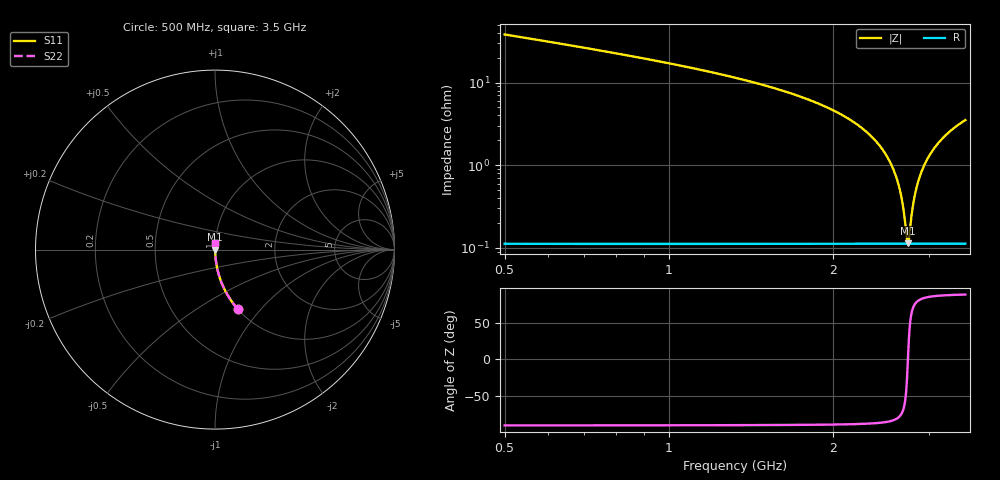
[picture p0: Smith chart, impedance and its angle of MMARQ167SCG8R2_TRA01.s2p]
! MMARQ167SCG8R2_TRA01  S-PARAMETER MODEL  ( General Type )
! Model Generated by TAIYO YUDEN Corporation (http://www.ty-top.com)
! Version 1.0
! TAIYO YUDEN Control No. 150305
! Copyright(c) 2015 TAIYO YUDEN CO.,LTD. All Rights Reserved.
! Product Description (link to TY-COMPAS)
! https://ds.yuden.co.jp/TYCOMPAS/or/detail?pn=MMARQ167SCG8R2CTRA01&u=M
! Products Name : Multilayer Ceramic Capacitors
! Characteristics :
!  Capacitance : 8.2 pF , Rated Voltage : 250V , TCC : CG / C0G
!  Case Size : 1.6 x 0.8 / 0.063 x 0.031 [mm/inch] , Thickness : 0.7 / 0.028 [mm/inch]
!  (Conditions: Temperature = 25 degC , DC Bias Current/Voltage = 0A / 0V)
! External Node Assignments :
!  1  o---| |---o  2
! GND o---------o GND
! Frequency Range : 500MHz  -  3.5GHz  [ 401 STEP ]
# MHz S RI R 50
! Freq[MHz].  S11 Real  S11 Imag  S21 Real  S21 Imag  S12 Real  S12 Imag  S22 Real  S22 Imag
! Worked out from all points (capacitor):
!   401 points, 500 MHz to 3.5 GHz, reference 50 ohm
!   read as one part in series: C = 8.06 pF near 515 MHz
!   lowest |Z| = 114 mohm at 2.743 GHz (marker M1)
!   series resonance near 2.746 GHz, so ESL is about 420 pH
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500  0.1281 -0.3327  0.8719 0.3327  0.8719 0.3327  0.1281 -0.3327
710  0.0641 -0.2427  0.9359 0.2427  0.9359 0.2427  0.0641 -0.2427
1002.5  0.0294 -0.1656  0.9706 0.1656  0.9706 0.1656  0.0294 -0.1656
1505  0.00945 -0.0909  0.9905 0.0909  0.9905 0.0909  0.00945 -0.0909
2000  0.00326 -0.0462  0.9967 0.0462  0.9967 0.0462  0.00326 -0.0462
2300  0.00177 -0.0256  0.9982 0.0256  0.9982 0.0256  0.00177 -0.0256
2412.5  0.00147 -0.0186  0.9985 0.0186  0.9985 0.0186  0.00147 -0.0186
2502.5  0.0013 -0.0133  0.9987 0.0133  0.9987 0.0133  0.0013 -0.0133
2585  0.0012 -0.00867  0.9988 0.00867  0.9988 0.00867  0.0012 -0.00867
2645  0.00115 -0.00537  0.9988 0.00537  0.9988 0.00537  0.00115 -0.00537
2682.5  0.00113 -0.00335  0.9989 0.00335  0.9989 0.00335  0.00113 -0.00335
2727.5  0.00112 -0.000958  0.9989 0.000958  0.9989 0.000958  0.00112 -0.000958
2742.5  0.00112 -0.00017  0.9989 0.00017  0.9989 0.00017  0.00112 -0.00017
2757.5  0.00112 0.000613  0.9989 -0.000613  0.9989 -0.000613  0.00112 0.000613
2802.5  0.00113 0.00294  0.9989 -0.00294  0.9989 -0.00294  0.00113 0.00294
2825  0.00114 0.00409  0.9989 -0.00409  0.9989 -0.00409  0.00114 0.00409
2855  0.00115 0.0056  0.9988 -0.0056  0.9988 -0.0056  0.00115 0.0056
2922.5  0.0012 0.00896  0.9988 -0.00896  0.9988 -0.00896  0.0012 0.00896
3005  0.00129 0.013  0.9987 -0.013  0.9987 -0.013  0.00129 0.013
3102.5  0.00143 0.0176  0.9986 -0.0176  0.9986 -0.0176  0.00143 0.0176
3215  0.00164 0.0227  0.9984 -0.0227  0.9984 -0.0227  0.00164 0.0227
3500  0.00236 0.0351  0.9976 -0.0351  0.9976 -0.0351  0.00236 0.0351
